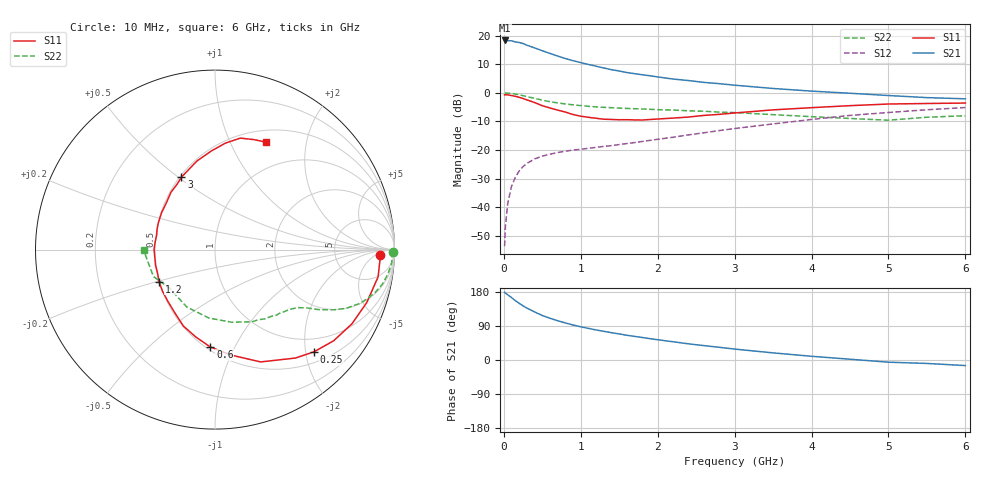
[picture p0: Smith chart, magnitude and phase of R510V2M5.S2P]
! SIEMENS Small Signal Semiconductors
! BFR183
! Si NPN RF Bipolar Junction Transistor in SOT23
! VCE = 10 V  IC = 2.5 mA
! Common Emitter S-Parameters:  May  1996
# GHz  S  MA  R  50
!  f  S11  S21  S12  S22
! GHz  MAG  ANG  MAG  ANG  MAG  ANG  MAG  ANG
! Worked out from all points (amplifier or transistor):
!   36 points, 10 MHz to 6 GHz, reference 50 ohm
!   highest |S21| = 18.3 dB at 10 MHz (marker M1)
!   |S21| within 3 dB of that: start of sweep to 440.6 MHz
!   unconditionally stable (mu >= 1): 1.351 GHz to 2.854 GHz
!   at 250 MHz: K = 0.26, MSG = 21.5 dB, |S12| = -25.8 dB
!   at 1.4 GHz: K = 1.02, MAG = 12.4 dB, |S12| = -18.4 dB
!   at 6 GHz: K = 0.88, MSG = 1.5 dB, |S12| = -5.2 dB
!   S11 on the Smith chart (normalised r, x): 10 MHz: 21, -9; 250 MHz: 0.71, -2.17; 600 MHz: 0.52, -0.81; 1.2 GHz: 0.50, -0.20; 3 GHz: 0.51, +0.51; 6 GHz: 0.64, +1.37
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0.01  0.9223 -1.9  8.201 178.5  0.0021 82.8  0.9932 -0.8
0.02  0.9205 -4.1  8.053 176.6  0.0046 83.8  0.9865 -1.6
0.05  0.9213 -9.5  8.11 172.2  0.0116 84.7  0.9881 -4.1
0.1  0.8956 -19.2  8.097 164.7  0.0233 79.2  0.9733 -8.1
0.15  0.868 -28.4  7.714 156.5  0.0336 73.9  0.9514 -11.8
0.2  0.8338 -37.5  7.558 149.6  0.0433 69.2  0.9235 -15.0
0.25  0.7931 -45.9  7.237 142.8  0.0515 65.5  0.8906 -18.0
0.3  0.7524 -53.4  6.763 137.0  0.0584 62.1  0.8584 -20.5
0.4  0.6754 -67.9  6.085 126.9  0.0701 56.6  0.801 -24.1
0.5  0.5949 -81.2  5.421 117.4  0.0784 52.6  0.7441 -26.8
0.6  0.5433 -92.7  4.87 110.1  0.0848 50.1  0.6989 -28.7
0.8  0.4609 -112.5  3.962 97.8  0.0955 46.8  0.6382 -31.1
0.9  0.4171 -122.5  3.636 92.3  0.1002 46.8  0.6168 -32.0
1.1  0.3732 -141.7  3.128 83.4  0.1075 47.2  0.5811 -33.9
1.2  0.3591 -150.2  2.913 79.3  0.1115 47.7  0.5677 -34.7
1.6  0.3394 179.7  2.259 65.2  0.1301 50.2  0.5333 -38.6
2.2  0.3617 145.5  1.738 48.1  0.1675 53.8  0.5006 -46.9
3  0.4444 114.9  1.358 28.8  0.2376 52.8  0.4518 -62.9
3.5  0.5035 101.6  1.19 18.8  0.2862 49.2  0.4153 -77.0
4.5  0.5962 84.4  0.982 2.1  0.403 38.5  0.3563 -116.1
5.5  0.6504 70.4  0.824 -9.1  0.5059 25.3  0.3743 -156.4
6  0.6622 64.8  0.785 -14.7  0.5525 16.5  0.3978 -179.5
